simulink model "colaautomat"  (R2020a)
settings: Solver=FixedStepDiscrete  StartTime=0.0  StopTime=30  RelTol=1e-3  EnableMultiTasking=on
libraries: simulink x3

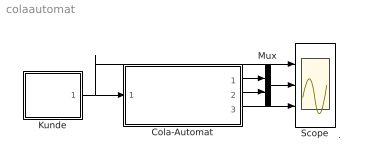
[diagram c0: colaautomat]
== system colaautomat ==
  note: .
  Cola-Automat : Subsystem  mask(Colaautomat){preis=220}
      mask prompts: preis "Dosenpreis"
      mask help: Modell fuer einen einfachen Colaautomaten.
  Kunde : Subsystem  mask(Kunde){p10=0.5, p50=0.2}
      mask prompts: p10 "Anteil 10er"; p50 "Anteil 50er"
      mask help: einfaches Kundenmodell: Der Kunde zieht wahllos Muenzen (10er, 50er, 100er) aus der Tasche.
  Mux : Mux  Inputs=2
  Scope : Scope  NumInputPorts=3
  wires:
  Kunde/1(Muenze) -> Cola-Automat/1(Muenzeinwurf), Scope/1
  Cola-Automat/1(Betrag) -> Mux/1
  Cola-Automat/2(Rueckgabe) -> Mux/2
  Mux/1 -> Scope/2
  Cola-Automat/3(Dosenauswurf) -> Scope/3

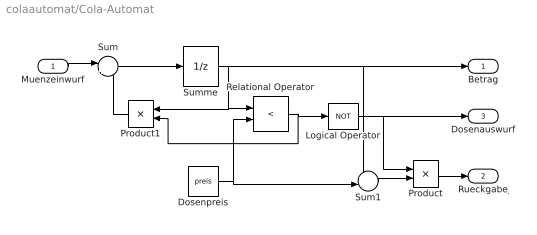
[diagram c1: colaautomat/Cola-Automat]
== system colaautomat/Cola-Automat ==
  note: .
  Muenzeinwurf : Inport
  Dosenpreis : Constant  Value=preis
  Logical Operator : Logic  Operator=NOT
  Product : Product  InputSameDT=on  SaturateOnIntegerOverflow=on
  Product1 : Product  InputSameDT=on  SaturateOnIntegerOverflow=on
  Relational Operator : RelationalOperator  Operator=<
  Sum : Sum  Inputs=|++  InputSameDT=on  SaturateOnIntegerOverflow=on
  Sum1 : Sum  Inputs=+-|  InputSameDT=on  SaturateOnIntegerOverflow=on
  Summe : UnitDelay  SampleTime=-1  HasFrameUpgradeWarning=on
  Betrag : Outport
  Rueckgabe : Outport  Port=2
  Dosenauswurf : Outport  Port=3
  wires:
  Summe/1 -> Betrag/1, Sum1/1, Relational Operator/1, Product1/1
  Dosenpreis/1 -> Relational Operator/2, Sum1/2
  Muenzeinwurf/1 -> Sum/1
  Relational Operator/1 -> Product1/2, Logical Operator/1
  Sum1/1 -> Product/2
  Product/1 -> Rueckgabe/1
  Sum/1 -> Summe/1
  Product1/1 -> Sum/2
  Logical Operator/1 -> Dosenauswurf/1, Product/1

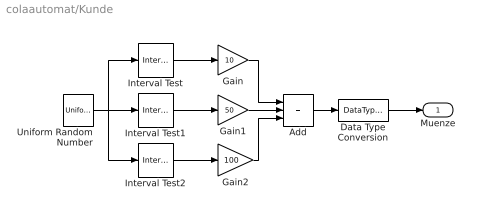
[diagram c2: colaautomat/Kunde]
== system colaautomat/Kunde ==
  note: .
  Add : Sum  Inputs=3
  Data Type Conversion : DataTypeConversion  OutDataTypeStr=double
  Gain : Gain  Gain=10
  Gain1 : Gain  Gain=50
  Gain2 : Gain  Gain=100
  Interval Test : simulink/Logic and Bit Operations/Interval Test  IntervalClosedRight=off  uplimit=p10  IntervalClosedLeft=on  lowlimit=0  OutDataTypeStr=uint8
  Interval Test1 : simulink/Logic and Bit Operations/Interval Test  IntervalClosedRight=off  uplimit=p10+p50  IntervalClosedLeft=on  lowlimit=p10  OutDataTypeStr=uint8
  Interval Test2 : simulink/Logic and Bit Operations/Interval Test  IntervalClosedRight=on  uplimit=1  IntervalClosedLeft=on  lowlimit=p10+p50  OutDataTypeStr=uint8
  Uniform Random Number : UniformRandomNumber  Minimum=0  SampleTime=1
  Muenze : Outport
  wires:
  Uniform Random Number/1 -> Interval Test1/1, Interval Test/1, Interval Test2/1
  Interval Test/1 -> Gain/1
  Interval Test1/1 -> Gain1/1
  Interval Test2/1 -> Gain2/1
  Gain/1 -> Add/1
  Gain1/1 -> Add/2
  Gain2/1 -> Add/3
  Add/1 -> Data Type Conversion/1
  Data Type Conversion/1 -> Muenze/1
